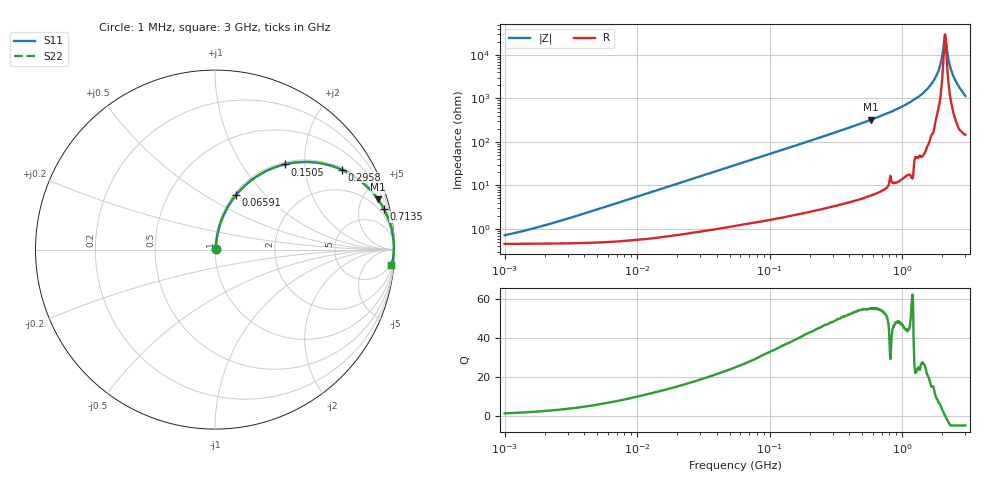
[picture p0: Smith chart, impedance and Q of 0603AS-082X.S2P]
!s-Parameter Generated by FASTRON Sdn. Bhd.
!FASTRON P/N : 0603AS-082X
!Keysight Technologies: E4991B_MY54100416_A.01.15
!Date created: Wed Oct 04 11:06:00 2023
!Version  : Rev01 Wed Oct 04 11:06:00 2023
!Data & Calibration Information:
!Freq	S11	S21	S12	S22
!PortZ  Port1:50+j0  Port2:50+j0
!When reading reference impedance value at option line is always used.
! Remarks : This data is being provided solely for informational purposes.
# Hz S dB R 50
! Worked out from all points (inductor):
!   1601 points, 1 MHz to 3 GHz, reference 50 ohm
!   read as one part in series: L = 88.3 nH near 2.499 MHz
!   highest Q = 55.3 at 581.2 MHz (marker M1), where L = 88.6 nH
!   self-resonance near 2.103 GHz
!   S11 on the Smith chart (normalised r, x): 1 MHz: 1.01, +0.01; 65.91 MHz: 1.03, +0.70; 150.5 MHz: 1.04, +1.58; 295.8 MHz: 1.06, +3.13; 713.5 MHz: 1.15, +8.27; 3 GHz: 4, -23
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1000000  -42.93 50.7  -0.04 -0.3  -0.04 -0.3  -42.93 50.7
3804036  -33.36 76.2  -0.04 -1.2  -0.04 -1.2  -33.36 76.2
1.447069e7  -22.11 80.9  -0.08 -4.5  -0.08 -4.5  -22.11 80.9
5.477226e7  -11.15 71.6  -0.45 -16.1  -0.45 -16.1  -11.15 71.6
6.591269e7  -9.72 68.8  -0.60 -19.0  -0.60 -19.0  -9.72 68.8
1.505037e8  -4.25 50.7  -2.22 -37.8  -2.22 -37.8  -4.25 50.7
2.083556e8  -2.73 41.7  -3.53 -46.9  -3.53 -46.9  -2.73 41.7
2.957531e8  -1.57 32.2  -5.46 -56.6  -5.46 -56.6  -1.57 32.2
5.81181e8  -0.44 17.1  -10.64 -71.9  -10.64 -71.9  -0.44 17.1
7.135306e8  -0.28 13.5  -12.61 -75.4  -12.61 -75.4  -0.28 13.5
7.925923e8  -0.23 11.8  -13.75 -76.9  -13.75 -76.9  -0.23 11.8
1.159346e9  -0.08 6.8  -18.54 -82.1  -18.54 -82.1  -0.08 6.8
1.621129e9  -0.04 2.9  -25.86 -83.8  -25.86 -83.8  -0.04 2.9
1.874306e9  -0.03 1.3  -32.61 -80.9  -32.61 -80.9  -0.03 1.3
1.960646e9  -0.03 0.8  -36.67 -77.5  -36.67 -77.5  -0.03 0.8
2.050964e9  -0.03 0.3  -43.98 -58.9  -43.98 -58.9  -0.03 0.3
2.102926e9  -0.03 0.0  -49.49 -8.4  -49.49 -8.4  -0.03 0.0
2.156205e9  -0.03 -0.3  -44.94 52.4  -44.94 52.4  -0.03 -0.3
2.278218e9  -0.03 -0.9  -35.74 75.9  -35.74 75.9  -0.03 -0.9
2.41921e9  -0.04 -1.6  -30.73 79.8  -30.73 79.8  -0.04 -1.6
2.673854e9  -0.06 -3.0  -25.63 80.8  -25.63 80.8  -0.06 -3.0
3e9  -0.13 -4.9  -21.27 77.7  -21.27 77.7  -0.13 -4.9
